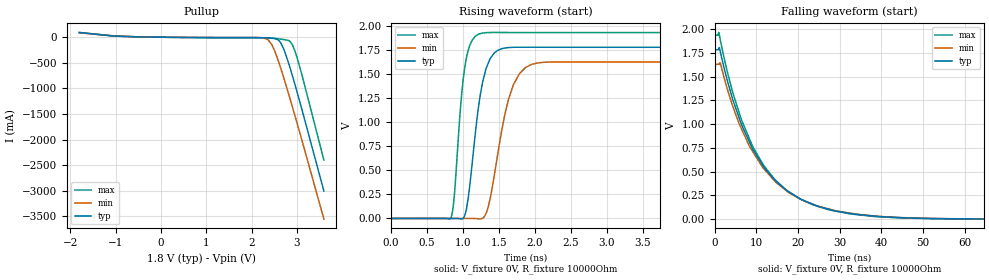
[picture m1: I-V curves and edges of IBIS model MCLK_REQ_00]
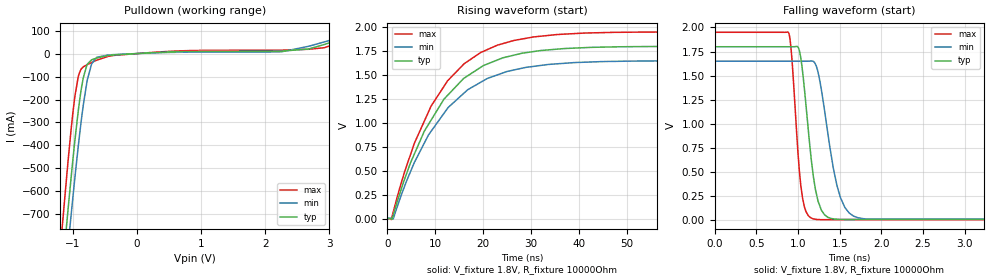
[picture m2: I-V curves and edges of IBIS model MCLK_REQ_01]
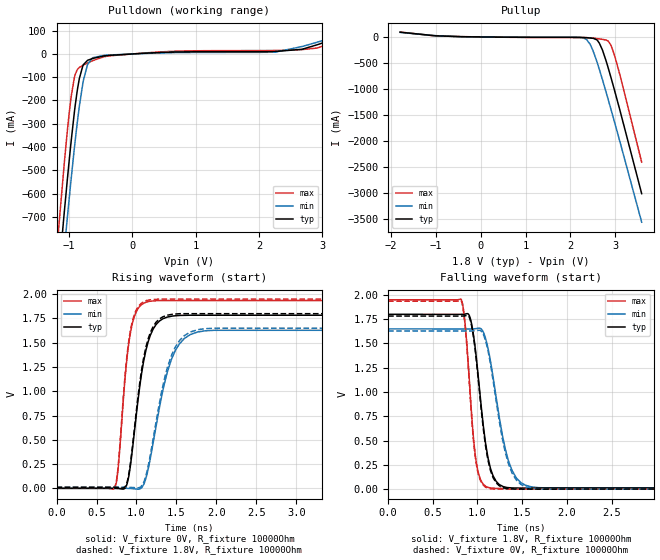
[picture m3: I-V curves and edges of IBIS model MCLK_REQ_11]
| Texas Instruments Incorporated
| Quad Sine-Wave Clock Buffer with LDO
| Marketing part#   Voltage Range   Package-type   #pins/pkg drawing
| CDC3S04YFFR   1.65V - 1.95V   WCSP   20-pin YFFR
| Package Dimension   Width   Length   Height
|   346.0mm   346.0mm   41.0mm
[IBIS ver]   4.0
[File name]   cdc3s04.ibs
[File Rev]   1.0
[Date]   08/29/2012
[Source]   Texas Instruments Incorporated.
   Analog-eLab, HPA
   12500 TI Blvd
   Dallas, TX -75243
   For Support e-mail: elab_ibis@list.ti.com
[Notes]   Revision History
   Rev 1.0: 12/16/2009
   - Initial version of the model
   - Model based on simulations from TIspiceD
   - Model not matched to measurements
   - min C_comp was obtained at corner high VDD, low  temperature, strong process
   - max C_comp was obtained at corner low  VDD, high temperature, weak process
   Rev 1.1: 01/11/2010
   - Pin assignment was not right.
   Rev 1.2: 08/29/2012
   - MCLK_REQ_xx regenerated.
   - Vmeas for SDAH_HS_X corrected.
   - Max corner temp changed to -40C.
   - Disclamimer section updated.
   - C_comp for TERM changed to 1fF.
   - POwer clmap non-mononitinicity of SDAH_HS_X corrected.
[Disclaimer]
  This model is designed as an aid for customers of Texas Instruments.
  TI and its licensors and suppliers make no warranties, either expressed
  or implied, with respect to this model, including the warranties of
  merchantability or fitness for a particular purpose.  The model is
  provided solely on an "as is" basis.  The entire risk as to its quality
  and performance is with the customer.
[Copyright] (C) Copyright 2012Texas Instruments Incorporated.
   All rights reserved.
|   Component CDC3S04
[Component]   CDC3S04
[Manufacturer]  Texas Instruments Incorporated
[Package]   |20-pin WCSP YFFR package
|   typ   min   max
R_pkg   20.50m   7.0m   80.0m
L_pkg   0.578nH   0.340nH   1.580nH
C_pkg   0.522pF   0.425pF   0.916pF
[Pin] signal_name   model_name   R_pin   L_pin   C_pin
|   Ohm   Henry   Farad
   A1  REQ2   REQ2_ibis   8m   0.368n   0.439p
   A2  CLK2   TERM   7m   0.340n   0.425p
   A3  REQ1   REQ1_ibis   9m   0.379n   0.441p
   A4  CLK1   TERM   10m   0.381n   0.433p
   B1  MCLK_IN   TERM   80m   1.580n   0.916p
   B2  RESET   NRESET_ibis   39m   0.942n   0.695p
   B3  VDD_ANA   POWER   11m   0.410n   0.453p
   B4  GND_ANA   GND   10m   0.397n   0.446p
   C1  REQ4   REQ4_ibis   39m   0.940n   0.694p
   C2  CLK4   TERM   10m   0.385n   0.434p
   C3  REQ3   REQ3_ibis   9m   0.371n   0.433p
   C4  CLK3   TERM   39m   0.920n   0.670p
   D1  VDD_DIG   POWER   10m   0.387n   0.435p
   D2  GND_DIG   GND   11m   0.395n   0.437p
   D3  MCLK_REQ   MCLK_REQ   38m   0.930n   0.690p
   D4  ADR_A0   ADR_A0_ibis   42m   0.941n   0.665p
   E1  VLD0   TERM   10m   0.384n   0.434p
   E2  VBAT   POWER   9m   0.361n   0.430p
   E3  SDAH   SDAH_HS   9m   0.369n   0.433p
   E4  SCLH   SCLH_HS   9m   0.374n   0.440p
[Pin Mapping] pulldown_ref pullup_ref gnd_clamp_ref power_clamp_ref
|   GNDBUS1 is GND_DIG,   PWRBUS1   is   VDD_DIG
A1   GNDBUS1   PWRBUS1   GNDBUS1   PWRBUS1  | input
A2   NC   NC   NC   NC   | analog output
A3   GNDBUS1   PWRBUS1   GNDBUS1   PWRBUS1  | input
A4   NC   NC   NC   NC   | analog output
B1   NC   NC   NC   NC   | analog input
B2   GNDBUS1   PWRBUS1   GNDBUS1   PWRBUS1  | input
B3   NC   PWRBUS2   | VDD_ANA
B4   GNDBUS2   NC   | VSS_ANA
C1   NC   PWRBUS1   | input
C2   NC   NC   NC   NC   | analog output
C3   GNDBUS1   PWRBUS1   GNDBUS1   PWRBUS1  | input
C4   NC   NC   NC   NC   | analog output
D1   NC   PWRBUS1   | power
D2   GNDBUS1   NC   | ground
D3   GNDBUS1   PWRBUS1   GNDBUS1   PWRBUS1  | output
D4   GNDBUS1   PWRBUS1   GNDBUS1   PWRBUS1  | input
E1   NC   NC   NC   NC   | analog output
E2   NC   PWRBUS3   | power
E3   GNDBUS1   PWRBUS1   GNDBUS1   PWRBUS1  | i/o
E4   GNDBUS1   PWRBUS1   GNDBUS1   PWRBUS1  | input
[Model Selector]   SCLH_HS
SCLH_HS_0   400KHz Input Model
SCLH_HS_1   3.4MHz Input Model
[Model Selector]   SDAH_HS
SDAH_HS_0   400KHz I/O Open-Sink Model
SDAH_HS_1   3.4MHz I/O Open-Sink Model
[Model Selector]   MCLK_REQ
MCLK_REQ_00   Output Open-Source Model
MCLK_REQ_01   Output Open-Sink Model
MCLK_REQ_11   1.65V - 1.95V Output Model
[Model] TERM
Model_type Terminator
C_comp   1fF  1fF  1fF
| variable   typ   min   max
[Voltage Range]   1.8000V   1.6500V   1.9500V
[power clamp reference]  1.8000V   1.6500V   1.9500V
[GND Clamp Reference]   0.00000V   0.0000V   0.0000V
[Temperature Range]   32   85   -40.0
| Models and submodels in the file (14): MCLK_REQ_00 (Open_source), MCLK_REQ_01 (Open_sink), MCLK_REQ_11 (Output), TERM (Terminator), ADR_A0_ibis (Input), NRESET_ibis (Input), REQ1_ibis (Input), REQ2_ibis (Input), REQ3_ibis (Input), REQ4_ibis (Input), SCLH_HS_0 (Input), SCLH_HS_1 (Input), SDAH_HS_0 (I/O_open_sink), SDAH_HS_1 (I/O_open_sink)
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|   1.8V-OUTPUT model
[Model]   MCLK_REQ_00
Model_type   Open_source
Polarity   Non-Inverting
Vmeas = 0.9
Vref = 0
Cref = 1pF
Rref = 10000
|   typ   min   max
C_comp   912.4fF   883.7fF   939.6fF
[Voltage Range]   1.8   1.65   1.95
[Temperature Range]   32   85   -40
[Pullup Reference]   1.8   1.65   1.95
[Pulldown Reference]   -0   -0   -0
[Power Clamp Reference]   1.8   1.65   1.95
[GND Clamp Reference]   -0   -0   -0
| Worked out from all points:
|   slope of the pullup table from 0 to 0.27 V, typ, clamps not added: 106 ohm
|   falling waveform, V_fixture 0V, R_fixture 10000Ohm: 20-80 % time 12.6ns typ, 13ns min, 12.1ns max; typ from 1.78 V to 0 V
|   rising waveform, V_fixture 0V, R_fixture 10000Ohm: 20-80 % time 178ps typ, 253ps min, 126ps max; typ from 0 V to 1.78 V
[Pullup]
|   Voltage   I(typ)   I(min)   I(max)
-1.8V     91.17mA    86.32mA    92.78mA
-1.001V   21.63mA    23.72mA    20.37mA
2.12V     -8.319mA   -6.671mA   -12mA
2.358V    -14.49mA   -43.3mA    -13.48mA
2.509V    -26.65mA   -267.9mA   -22.98mA
2.65V     -120.1mA   -624.5mA   -38.19mA
2.725V    -268.3mA   -839.7mA   -47.83mA
2.833V    -555mA     -1.16A     -72.68mA
2.909V    -779.2mA   -1.39A     -164mA
2.99V     -1.03A     -1.639A    -360.9mA
3.109V    -1.407A    -2.01A     -727.4mA
3.595V    -3.008A    -3.555A    -2.403A
[Ramp]
R_load = 10000
|   typ   min   max
dV/dt_r   1.06946/1.77831e-10   0.977333/2.53409e-10   1.16133/1.25521e-10
dV/dt_f   1.06946/1.25771e-08   0.977333/1.29607e-08   1.16133/1.21188e-08
[Falling Waveform]
V_fixture = 0V
V_fixture_min = 0V
V_fixture_max = 0V
R_fixture = 10000Ohm
C_fixture = 0F
|   Time   V(typ)   V(min)   V(max)
0s        1.782V     1.629V     1.936V
985.8ps   1.791V     1.629V     1.963V
1.353ns   1.76V      1.641V     1.883V
3.058ns   1.453V     1.364V     1.544V
6.433ns   994.7mV    949.5mV    1.043V
11.74ns   552.2mV    532.5mV    565.5mV
17.04ns   310.4mV    304.9mV    310.5mV
23.44ns   158.4mV    157.9mV    152mV
45.59ns   12.51mV    14.34mV    11.17mV
100ns     -7.067uV   8.797uV    -4.691uV
[Rising Waveform]
V_fixture = 0V
V_fixture_min = 0V
V_fixture_max = 0V
R_fixture = 10000Ohm
C_fixture = 0F
|   Time   V(typ)   V(min)   V(max)
0s        -7.059uV   8.797uV    -4.691uV
833.8ps   233.3uV    7.746uV    5.77mV
873.4ps   244.8uV    7.697uV    175.2mV
971.6ps   -4.911mV   7.573uV    1.193V
1.047ns   88.56mV    105.4uV    1.665V
1.213ns   1.136V     -2.974mV   1.916V
1.335ns   1.584V     78.79mV    1.935V
1.7ns     1.782V     1.388V     1.936V
2.233ns   1.783V     1.629V     1.935V
100ns     1.782V     1.629V     1.936V
[Model]   MCLK_REQ_01
Model_type   Open_sink
Polarity   Non-Inverting
Vmeas = 0.9
Vref = 1.8
Cref = 1pF
Rref = 10000
|   typ   min   max
C_comp   945.8fF   920.5fF   972.8fF
[Voltage Range]   1.8   1.65   1.95
[Temperature Range]   32   85   -40
[Pullup Reference]   1.8   1.65   1.95
[Pulldown Reference]   -0   -0   -0
[Power Clamp Reference]   1.8   1.65   1.95
[GND Clamp Reference]   -0   -0   -0
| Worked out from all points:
|   slope of the pulldown table from 0 to 0.27 V, typ, clamps not added: 64.8 ohm
|   falling waveform, V_fixture 1.8V, R_fixture 10000Ohm: 20-80 % time 133ps typ, 188ps min, 93.3ps max; typ from 1.8 V to 0.01 V
|   rising waveform, V_fixture 1.8V, R_fixture 10000Ohm: 20-80 % time 12.2ns typ, 12.6ns min, 11.9ns max; typ from 0.01 V to 1.8 V
[Pulldown]
|   Voltage   I(typ)   I(min)   I(max)
-1.8V     -3.017A    -3.087A    -2.942A
-1.179V   -989.5mA   -1.143A    -790.2mA
-1.076V   -677.4mA   -839.1mA   -466.9mA
-1.028V   -536.4mA   -699.9mA   -327.3mA
-968.4mV  -374.2mA   -536mA     -183.4mA
-919.8mV  -255.1mA   -409.6mA   -104.3mA
-838.8mV  -105.1mA   -224mA     -57.91mA
-774mV    -45.58mA   -112.3mA   -47.49mA
-709.2mV  -27.28mA   -45.05mA   -38.76mA
-450mV    -8.568mA   -6.142mA   -12.04mA
2.682V    20.15mA    31.97mA    18.76mA
3.595V    101.6mA    105.5mA    92.12mA
[Ramp]
R_load = 10000
|   typ   min   max
dV/dt_r   1.07382/1.22312e-08   0.982408/1.26413e-08   1.16499/1.19181e-08
dV/dt_f   1.07382/1.326e-10   0.982408/1.88068e-10   1.16499/9.32535e-11
[Falling Waveform]
V_fixture = 1.8V
V_fixture_min = 1.65V
V_fixture_max = 1.95V
R_fixture = 10000Ohm
C_fixture = 0F
|   Time   V(typ)   V(min)   V(max)
0s        1.8V       1.65V      1.95V
885.2ps   1.8V       1.65V      1.949V
926.4ps   1.8V       1.65V      1.682V
1ns       1.796V     1.65V      697.2mV
1.055ns   1.544V     1.65V      231mV
1.184ns   457.8mV    1.648V     15.95mV
1.269ns   132.1mV    1.411V     7.729mV
1.509ns   10.09mV    236mV      8.154mV
1.865ns   10.12mV    13.15mV    8.374mV
100ns     10.27mV    12.6mV     8.348mV
[Rising Waveform]
V_fixture = 1.8V
V_fixture_min = 1.65V
V_fixture_max = 1.95V
R_fixture = 10000Ohm
C_fixture = 0F
|   Time   V(typ)   V(min)   V(max)
0s        10.27mV    12.6mV     8.348mV
815.4ps   10.43mV    12.72mV    -2.219mV
1.228ns   44.43mV    8.3mV      77.64mV
5.679ns   685.4mV    596.5mV    796.9mV
9.142ns   1.033V     917.1mV    1.179V
11.83ns   1.252V     1.104V     1.385V
15.94ns   1.466V     1.311V     1.614V
22.99ns   1.658V     1.504V     1.813V
39.2ns    1.783V     1.632V     1.933V
100ns     1.8V       1.65V      1.95V
[Model]   MCLK_REQ_11
Model_type   Output
Polarity   Non-Inverting
Vmeas = 0.9
Vref = 0
Cref = 1pF
Rref = 10000
|   typ   min   max
C_comp   945.8fF   920.5fF   972.8fF
[Voltage Range]   1.8   1.65   1.95
[Temperature Range]   32   85   -40
[Pullup Reference]   1.8   1.65   1.95
[Pulldown Reference]   -0   -0   -0
[Power Clamp Reference]   1.8   1.65   1.95
[GND Clamp Reference]   -0   -0   -0
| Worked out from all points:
|   slope of the pulldown table from 0 to 0.27 V, typ, clamps not added: 64.8 ohm
|   slope of the pullup table from 0 to 0.27 V, typ, clamps not added: 106 ohm
|   falling waveform, V_fixture 1.8V, R_fixture 10000Ohm: 20-80 % time 133ps typ, 188ps min, 94.4ps max; typ from 1.8 V to 0.01 V
|   rising waveform, V_fixture 0V, R_fixture 10000Ohm: 20-80 % time 176ps typ, 250ps min, 124ps max; typ from 0 V to 1.78 V
|   rising waveform, V_fixture 1.8V, R_fixture 10000Ohm: 20-80 % time 174ps typ, 246ps min, 123ps max; typ from 0.01 V to 1.8 V
|   falling waveform, V_fixture 0V, R_fixture 10000Ohm: 20-80 % time 131ps typ, 184ps min, 93.6ps max; typ from 1.78 V to 0 V
[Pulldown]
|   Voltage   I(typ)   I(min)   I(max)
-1.8V     -3.017A    -3.087A    -2.942A
-1.179V   -989.5mA   -1.143A    -790.2mA
-1.076V   -677.4mA   -839.1mA   -466.9mA
-1.028V   -536.4mA   -699.9mA   -327.3mA
-968.4mV  -374.2mA   -536mA     -183.4mA
-919.8mV  -255.1mA   -409.6mA   -104.3mA
-838.8mV  -105.1mA   -224mA     -57.91mA
-774mV    -45.58mA   -112.3mA   -47.49mA
-709.2mV  -27.28mA   -45.05mA   -38.76mA
-450mV    -8.568mA   -6.142mA   -12.04mA
2.682V    20.15mA    31.97mA    18.76mA
3.595V    101.6mA    105.5mA    92.12mA
[Pullup]
|   Voltage   I(typ)   I(min)   I(max)
-1.8V     91.17mA    86.32mA    92.78mA
-1.001V   21.63mA    23.72mA    20.37mA
2.12V     -8.319mA   -6.671mA   -12mA
2.358V    -14.49mA   -43.3mA    -13.48mA
2.509V    -26.65mA   -267.9mA   -22.98mA
2.65V     -120.1mA   -624.5mA   -38.19mA
2.725V    -268.3mA   -839.7mA   -47.83mA
2.833V    -555mA     -1.16A     -72.68mA
2.909V    -779.2mA   -1.39A     -164mA
2.99V     -1.03A     -1.639A    -360.9mA
3.109V    -1.407A    -2.01A     -727.4mA
3.595V    -3.008A    -3.555A    -2.403A
[Ramp]
R_load = 10000
|   typ   min   max
dV/dt_r   1.06946/1.76343e-10   0.977338/2.50029e-10   1.16132/1.24299e-10
dV/dt_f   1.07384/1.33117e-10   0.982437/1.87662e-10   1.16499/9.44007e-11
[Falling Waveform]
V_fixture = 1.8V
V_fixture_min = 1.65V
V_fixture_max = 1.95V
R_fixture = 10000Ohm
C_fixture = 0F
|   Time   V(typ)   V(min)   V(max)
0s        1.8V       1.65V      1.95V
818.8ps   1.8V       1.65V      1.952V
867ps     1.804V     1.65V      1.652V
920.2ps   1.757V     1.65V      960.9mV
1ns       1.24V      1.655V     206.3mV
1.117ns   324.7mV    1.454V     18.06mV
1.211ns   77.14mV    932.2mV    7.612mV
1.386ns   11.26mV    193.4mV    7.743mV
1.764ns   9.869mV    12mV       8.376mV
100ns     10.27mV    12.6mV     8.348mV
[Rising Waveform]
V_fixture = 0V
V_fixture_min = 0V
V_fixture_max = 0V
R_fixture = 10000Ohm
C_fixture = 0F
|   Time   V(typ)   V(min)   V(max)
0s        14.35nV    43.25nV    1.793nV
728.6ps   -167.3uV   120.3uV    6.228mV
772.7ps   -2.004mV   127.5uV    226.4mV
866.1ps   12.99mV    55.01uV    1.22V
955.7ps   448.3mV    -3.59mV    1.722V
1.092ns   1.319V     42.45mV    1.908V
1.274ns   1.713V     773.7mV    1.935V
1.536ns   1.781V     1.488V     1.935V
1.968ns   1.783V     1.628V     1.935V
100ns     1.782V     1.629V     1.936V
[Rising Waveform]
V_fixture = 1.8V
V_fixture_min = 1.65V
V_fixture_max = 1.95V
R_fixture = 10000Ohm
C_fixture = 0F
|   Time   V(typ)   V(min)   V(max)
0s        10.27mV    12.6mV     8.348mV
728.6ps   10.1mV     12.69mV    15.53mV
772.7ps   8.273mV    12.7mV     243.5mV
855.9ps   13.83mV    12.71mV    1.153V
985.2ps   699mV      6.638mV    1.816V
1.117ns   1.452V     128.2mV    1.932V
1.274ns   1.735V     821mV      1.949V
1.536ns   1.799V     1.52V      1.949V
1.968ns   1.799V     1.65V      1.949V
100ns     1.8V       1.65V      1.95V
[Falling Waveform]
|Gnd
V_fixture = 0V
V_fixture_min = 0V
V_fixture_max = 0V
R_fixture = 10000Ohm
C_fixture = 0F
|   Time   V(typ)   V(min)   V(max)
0s        1.782V     1.629V     1.936V
818.8ps   1.782V     1.629V     1.937V
867ps     1.786V     1.629V     1.635V
920.2ps   1.738V     1.629V     935.3mV
1ns       1.212V     1.634V     190mV
1.103ns   376.7mV    1.485V     14.27mV
1.211ns   62.21mV    892.7mV    -727.6uV
1.386ns   792.5uV    166.6mV    -576.2uV
1.764ns   -374.8uV   -672.5uV   27.52uV
100ns     14.35nV    43.25nV    1.793nV
